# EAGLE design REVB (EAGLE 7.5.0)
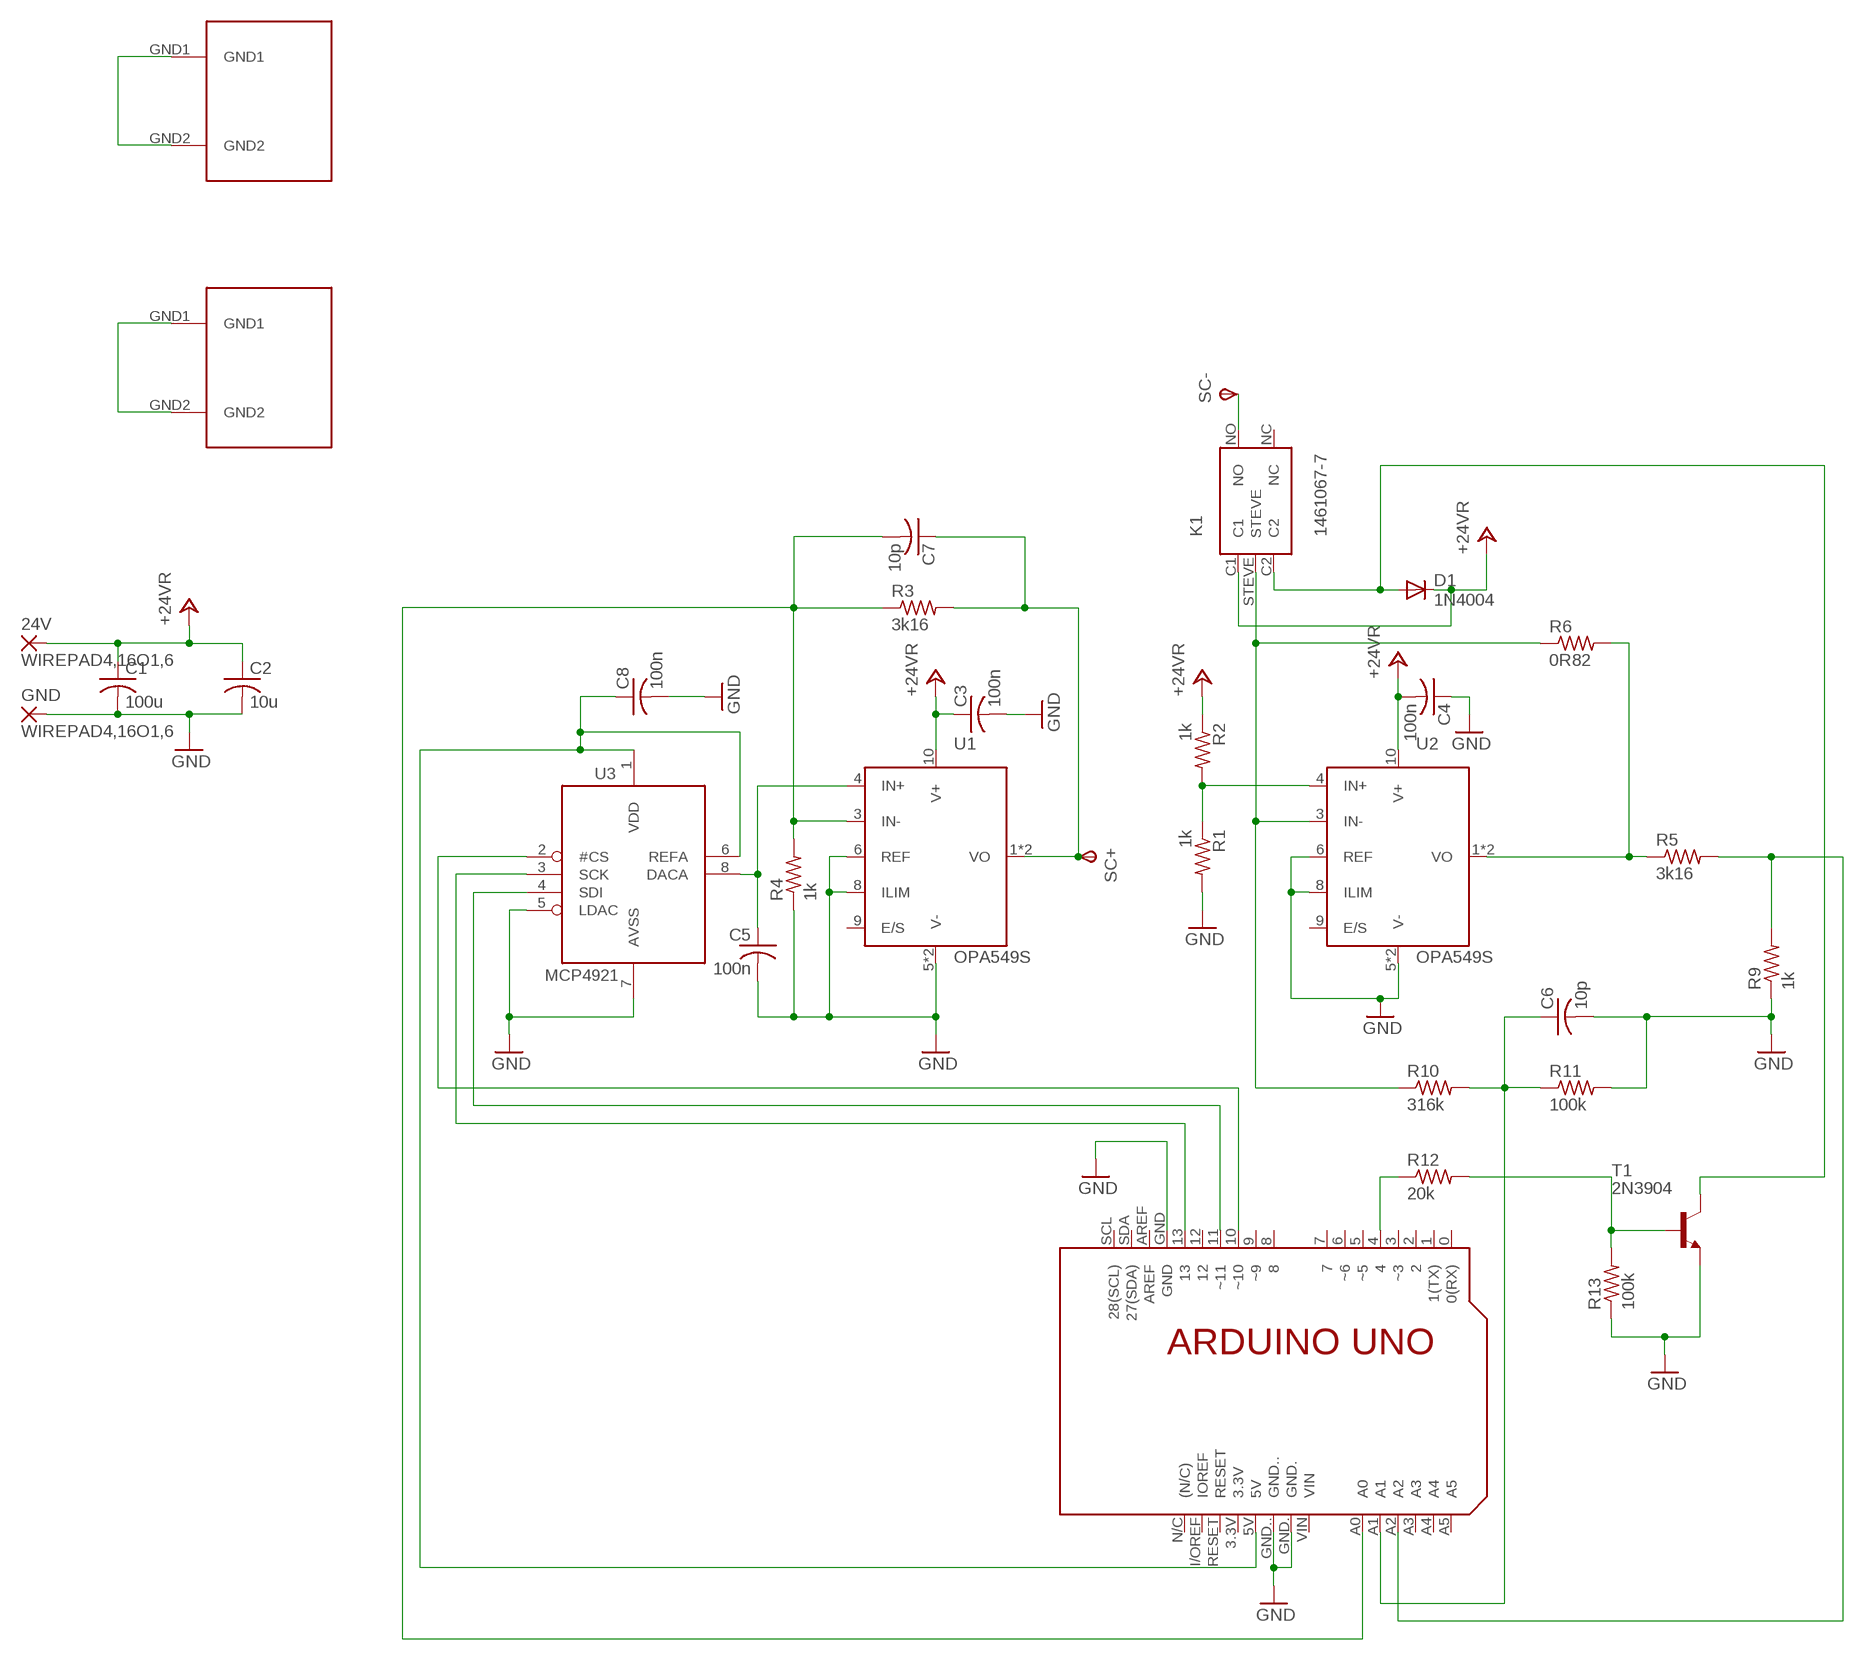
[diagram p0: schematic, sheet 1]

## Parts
24V  WIREPAD4,16O1,6  [4,16O1,6]
C1  100u  C-US050-050X075  [C050-050X075]
C2  10u  C-US025-024X044  [C025-024X044]
C3  100n  C-US025-024X044  [C025-024X044]
C4  100n  C-US025-024X044  [C025-024X044]
C5  100n  C-US025-024X044  [C025-024X044]
C6  10p  C-US025-024X044  [C025-024X044]
C7  10p  C-US025-024X044  [C025-024X044]
C8  100n  C-US025-024X044  [C025-024X044]
D1  1N4004  [DO41-10]
GND  WIREPAD4,16O1,6  [4,16O1,6]
K1  1461067-7  [1461067-7]
PCB1  ARDUINO_UNO  [ARDUINO_UNO]
R1  1k  R-US_0207/10  [0207/10]
R2  1k  R-US_0207/10  [0207/10]
R3  3k16  R-US_0207/10  [0207/10]
R4  1k  R-US_0207/10  [0207/10]
R5  3k16  R-US_0207/10  [0207/10]
R6  0R82  RESHS50  [HS50]
R9  1k  R-US_0207/10  [0207/10]
R10  316k  R-US_0207/10  [0207/10]
R11  100k  R-US_0207/10  [0207/10]
R12  20k  R-US_0207/10  [0207/10]
R13  100k  R-US_0207/10  [0207/10]
SC+  TPSPAD1-20  [P1-20]
SC-  TPSPAD1-20  [P1-20]
T1  2N3904  [TO92]
U1  OPA549S  [11TO-220]
U2  OPA549S  [11TO-220]
U3  MCP4921  [DIL08]
U$7  RA-T2X-64E  [RA-T2X-64E]
U$8  RA-T2X-64E  [RA-T2X-64E]

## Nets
+24V: 24V.1(P) C1.1 C2.1 C3.1 C4.2 D1.C K1.C1 R2.1 U1.10(V+) U2.10(V+) ; supply symbol labelled +24VR
GND: C1.2 C2.2 C3.2 C4.1 C5.2 C6.2 C8.2 GND.1(P) PCB1.GND PCB1.GND. PCB1.GND.. R1.2 R4.1 R9.1 R11.2 R13.1 T1.3(E) U1.5(V-) U1.6(REF) U1.7(V-) U1.8(ILIM) U2.5(V-) U2.6(REF) U2.7(V-) U2.8(ILIM) U3.5(LDAC) U3.7(AVSS)
ISO1: U$8.GND1 U$8.GND2
ISO2: U$7.GND1 U$7.GND2
N$1: C7.1 R3.2 SC+.TP(PP) U1.1(VO) U1.2(VO)
N$2: PCB1.10(~10) U3.2(#CS)
N$3: PCB1.13 U3.3(SCK)
N$4: PCB1.11(~11) U3.4(SDI)
N$5: R5.1 R6.P2 U2.1(VO) U2.2(VO)
N$6: C5.1 U1.4(IN+) U3.8(DACA)
N$7: C7.2 PCB1.A0 R3.1 R4.2 U1.3(IN-)
N$8: K1.NO SC-.TP(PP)
N$10: PCB1.A2 R5.2 R9.2
N$11: C6.1 PCB1.A1 R10.2 R11.1
N$12: PCB1.4 R12.1
N$13: R12.2 R13.2 T1.2(B)
N$14: D1.A K1.C2 T1.1(C)
N$26: K1.STEVE R6.P1 R10.1 U2.3(IN-)
N$31: R1.1 R2.2 U2.4(IN+)
VDD: C8.1 PCB1.5V U3.1(VDD) U3.6(REFA)
Unconnected: K1.NC PCB1.0(0(RX)) PCB1.1(1(TX)) PCB1.2 PCB1.3(~3) PCB1.3.3V PCB1.5(~5) PCB1.6(~6) PCB1.7 PCB1.8 PCB1.9(~9) PCB1.12 PCB1.A3 PCB1.A4 PCB1.A5 PCB1.AREF PCB1.I/OREF(IOREF) PCB1.N/C((N/C)) PCB1.RESET PCB1.SCL(28(SCL)) PCB1.SDA(27(SDA)) PCB1.VIN U1.9(E/S) U2.9(E/S)

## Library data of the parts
24V GND = wirepad:WIREPAD: Wire PAD connect wire on PCB
C1-C8 = rcl:C-US: CAPACITOR, American symbol
D1 = diode:1N4004: DIODE
K1 = aaron:1461067-7
PCB1 = E14_Arduino_revB:ARDUINO_UNO: Device for representing an Arduino Uno board with a footprint in an EAGLE design. Created by Dave Young for Element14. More EAGLE documentation at: http://www.element14.com/community/community/knode/cadsoft_eagle
R1-R5 R9-R13 = resistor:R-US_: RESISTOR, American symbol
R6 = aaron:RES
SC+ SC- = testpad:TPS: TEST PIN
T1 = transistor:2N3904: NPN TRANSISTOR
U1 U2 = aaron:OPA549S
U3 = adafruit:MCP4921
U$7 U$8 = DanECE4901:RA-T2X-64E

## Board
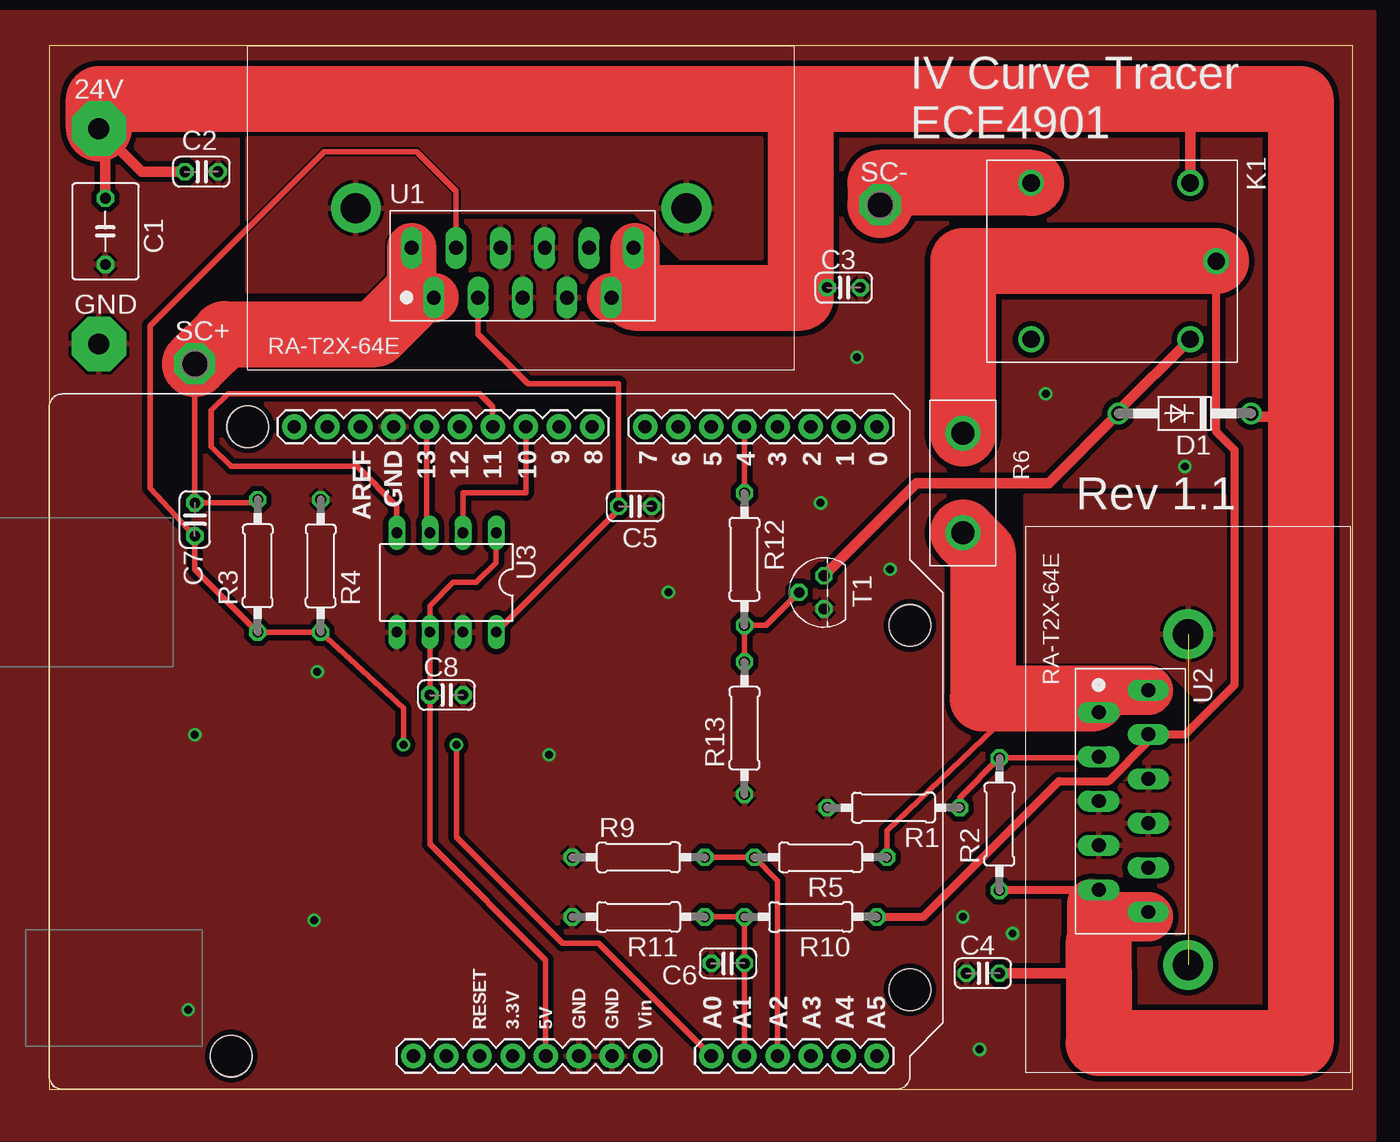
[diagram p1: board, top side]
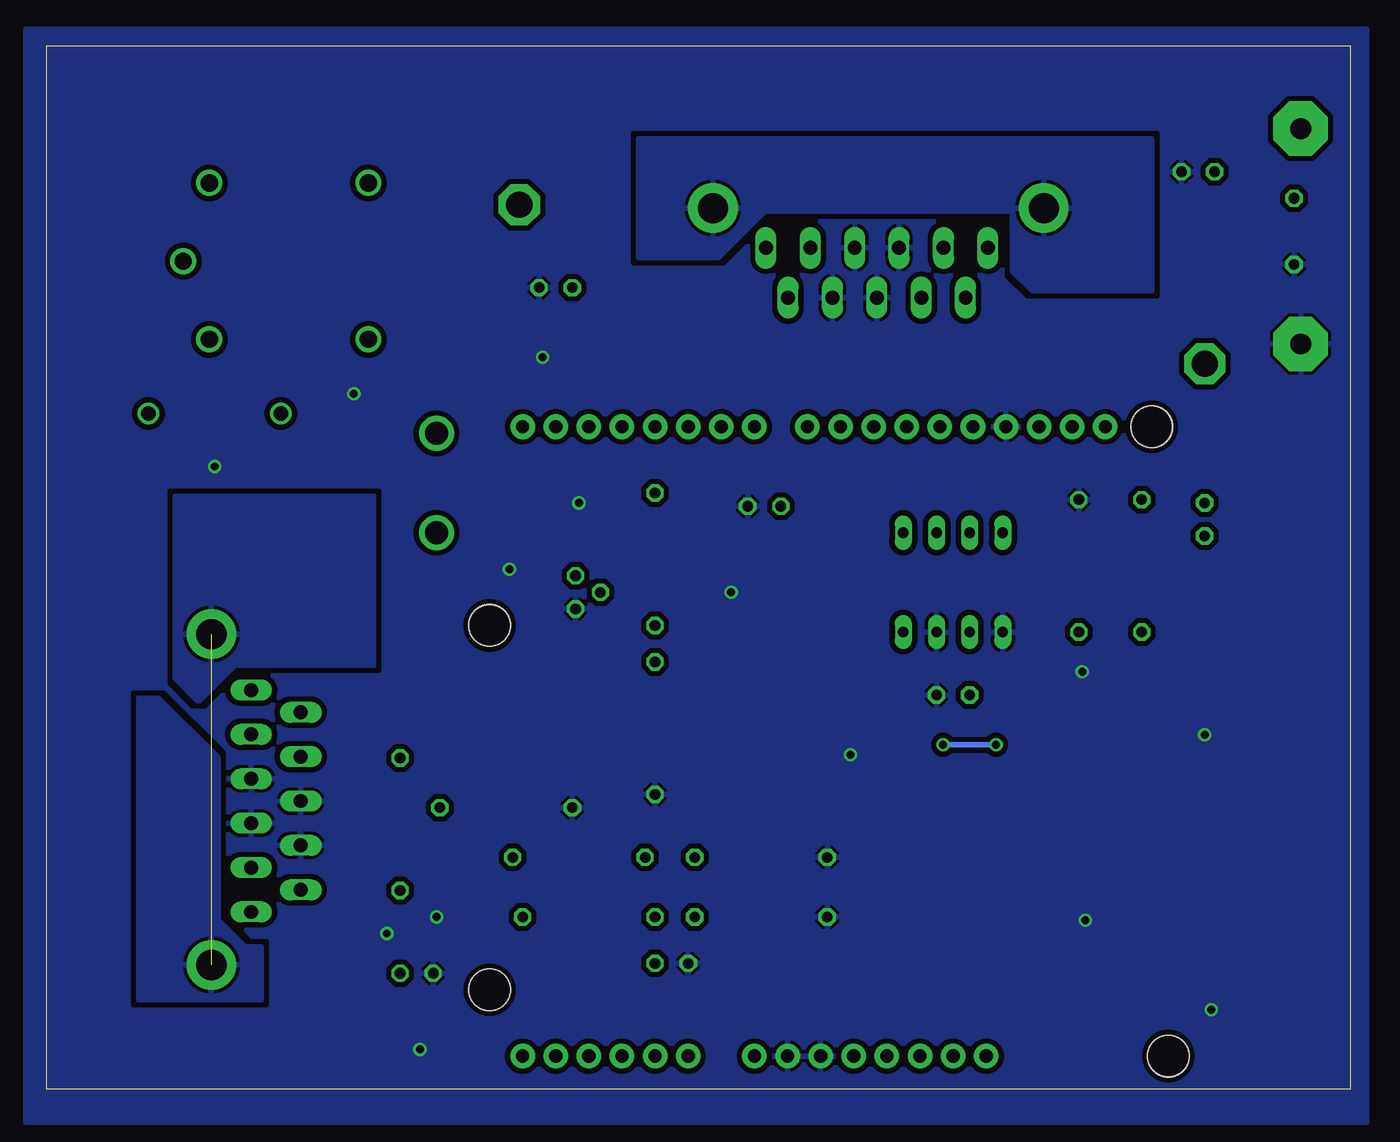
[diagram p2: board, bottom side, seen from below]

No outline drawn. Coordinates in mm, seen from the top.
Copper layers (1*16): Top 0.035559375mm / dielectric 1.501140625mm / Bottom 0.035559375mm
Design rules "typical_4pcb": minimum track width 10mil, minimum drill 15mil, track to track 6mil, track to pad 6mil, pad to pad 6mil, via to via 6mil, smd to smd 6mil, copper to edge 15mil, drill to drill 8mil, minimum pad ring 10mil, minimum via ring 8mil, stop-mask expansion 4mil, vias tented up to drill 0mil, thermal gap 10mil
Holes 3.17 mm at 15.24,50.8 66.04,35.56 66.04,7.62 13.97,2.54
Milling: 4 lines

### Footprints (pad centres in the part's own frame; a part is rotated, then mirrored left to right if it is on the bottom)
4,16O1,6 = drill 1.6 pad 4.166 octagon: 1 0,0
C050-050X075 = drill 0.813 octagon: 1 -2.54,0; 2 2.54,0
C025-024X044 = drill 0.813 octagon: 1 -1.27,0; 2 1.27,0
DO41-10 = drill 1.118: A 5.08,0; C -5.08,0
1461067-7 = drill 1.321: C1 6,6; C2 6,-6; NC -6.2,-6; NO -6.2,6; STEVE 8,0
ARDUINO_UNO = drill 1.016 pad 1.88: 0 63.5,50.8; 1 60.96,50.8; 2 58.42,50.8; 3 55.88,50.8; 3.3V 35.56,2.54; 4 53.34,50.8; 5 50.8,50.8; 5V 38.1,2.54; 6 48.26,50.8; 7 45.72,50.8; 8 41.656,50.8; 9 39.116,50.8; 10 36.576,50.8; 11 34.036,50.8; 12 31.496,50.8; 13 28.956,50.8; A0 50.8,2.54; A1 53.34,2.54; A2 55.88,2.54; A3 58.42,2.54; A4 60.96,2.54; A5 63.5,2.54; AREF 23.876,50.8; GND 26.416,50.8; GND. 43.18,2.54; GND.. 40.64,2.54; I/OREF 30.48,2.54; N/C 27.94,2.54; RESET 33.02,2.54; SCL 18.796,50.8; SDA 21.336,50.8; VIN 45.72,2.54 | hole 3.2: 66.04,7.62; 66.04,35.56; 15.24,50.8; 13.97,2.54
0207/10 = drill 0.813 octagon: 1 -5.08,0; 2 5.08,0
HS50 = drill 1.778: P1 -3.81,0; P2 3.81,0
P1-20 = drill 2.007 pad 3.15 octagon: TP 0,0
TO92 = drill 0.813 octagon: 1 1.27,0; 2 0,1.905; 3 -1.27,0
11TO-220 = drill 1.067 long: 1 -8.509,0; 2 -6.807,-3.81; 3 -5.105,0; 4 -3.404,-3.81; 5 -1.702,0; 6 0,-3.81; 7 1.702,0; 8 3.404,-3.81; 9 5.105,0; 10 6.807,-3.81; 11 8.509,0
DIL08 = drill 0.813 long: 1 -3.81,-3.81; 2 -1.27,-3.81; 3 1.27,-3.81; 4 3.81,-3.81; 5 3.81,3.81; 6 1.27,3.81; 7 -1.27,3.81; 8 -3.81,3.81
RA-T2X-64E = drill 2.311 pad 3.81: GND1 8.28,12.446; GND2 33.655,12.446

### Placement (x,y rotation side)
24V  3.81,73.66 0 top
C1  4.32,65.79 270 top
C2  11.68,70.36 0 top
C3  60.96,61.47 0 top
C4  71.63,8.89 0 top
C5  44.96,44.7 0 top
C6  52.07,9.65 180 top
C7  11.18,43.69 270 top
C8  30.48,30.23 0 top
D1  87.12,51.82 180 top
GND  3.81,57.15 0 top
K1  81.53,63.5 0 top
PCB1  0,0 0 top
R1  64.77,21.59 180 top
R2  72.9,20.32 90 top
R3  16,40.13 90 top
R4  20.83,40.13 270 top
R5  59.18,17.78 180 top
R6  70.1,46.48 270 top
R9  45.21,17.78 0 top
R10  58.42,13.21 180 top
R11  45.21,13.21 180 top
R12  53.34,40.64 270 top
R13  53.34,27.69 90 top
SC+  11.18,55.63 0 top
SC-  63.75,67.82 0 top
T1  59.44,38.1 90 top
U1  36.32,64.52 0 top
U2  84.33,22.1 270 top
U3  30.48,38.86 180 top
U$7  74.93,43.18 270 top
U$8  15.24,55.12 0 top

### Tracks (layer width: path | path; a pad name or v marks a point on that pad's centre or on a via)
+24V
  Top 0.305: 80.01,14.22 80.52,14.73 U2.10
  Top 0.406: 80.01,8.89 80.52,8.89 80.52,9.14 | 87.63,74.42 87.63,75.95
  Top 0.61: 57.66,60.71 58.93,60.71 C3.1 57.4,63.75 57.4,75.95 | R2.1 72.95,15.29 U2.10
  Top 0.813: C4.2 80.01,8.89 | D1.C 92.2,51.56 96.01,51.56 | 3.3,73.15 24V.1 | C1.1 4.32,73.15 24V.1 | C2.1 7.11,70.36 24V.1 | K1.C1 87.53,75.95 88.14,75.95
  Top 3.81: U1.10 44.96,60.71 44.96,64.52 | 80.52,11.18 80.01,11.68 80.01,14.22 81.03,13.21 84.33,13.21
  Top 5.08: 24V.1 3.81,75.95 57.4,75.95 87.63,75.95 88.14,75.95 96.01,75.95 96.01,51.56 96.01,3.56 80.52,3.56 80.52,9.14 80.52,11.18 | 44.96,60.71 57.66,60.71 57.66,73.91
GND  (via drill 0.6, 0.61)
  other vias: 87.12,47.75 11.18,27.18 20.32,12.95 10.67,6.1 47.5,38.1 38.35,25.65 70.1,13.21 73.91,11.94 76.45,53.34 59.18,44.96 64.52,39.88 71.37,3.05 20.57,32 61.98,56.13
  pour Top (isolate 0.406, rank 3): -3.81,82.55 101.6,82.55 101.6,-3.81 -3.81,-3.81
  pour Bottom (isolate 0.406, rank 3): -1.27,81.28 101.6,81.28 101.6,-2.54 -1.27,-2.54
ISO1
  pour Bottom: 54.61,72.9 15.24,72.9 15.24,61.21 24.38,61.21 25.91,62.74 25.91,67.31 44.96,67.31 48.51,63.75 54.61,63.75
  pour Top: 54.61,72.9 15.24,72.9 15.24,61.21 24.38,61.21 25.91,62.74 25.91,67.31 44.96,67.31 48.51,63.75 54.61,63.75
ISO2  (1 unrouted)
  pour Bottom: 90.17,45.47 74.93,45.47 74.93,32.51 85.6,32.51 88.39,29.72 90.17,31.5
  pour Top: 90.17,45.47 74.93,45.47 74.93,32.51 85.6,32.51 88.39,29.72 90.17,31.5
  pour Bottom: 83.57,6.86 92.96,6.86 92.96,29.97 91.44,29.97 86.87,25.4 86.87,12.95 84.84,10.92 83.57,10.92
N$1
  Top 0.406: R3.2 16,44.96 C7.1 SC+.TP
  Top 3.81: U1.1 27.81,60.71 U1.2
  Top 5.08: SC+.TP 13.46,57.91 25.02,57.91 27.81,60.71
N$2
  Top 0.406: PCB1.10 36.58,45.72 31.75,45.72 U3.2
N$3
  Top 0.406: PCB1.13 28.96,42.67 U3.3
N$4
  Top 0.406: PCB1.11 34.04,52.32 33.02,53.34 13.72,53.34 12.45,52.07 12.45,49.28 13.97,47.75 23.62,47.75 26.67,44.7 U3.4
N$5
  Top 0.406: R5.1 64.26,19.81 74.93,29.97
  Top 1.778: U2.2 80.52,30.48 | 80.52,30.48 79.5,30.61 | 80.01,29.97 79.5,30.48 80.52,30.48
  Top 3.81: U2.1 79.5,30.61
  Top 5.08: R6.P2 71.63,41.15 71.63,29.97 74.93,29.97 80.01,29.97
N$6
  Top 0.406: U3.8 43.69,44.45 C5.1 43.69,54.1 36.73,54.1 32.92,57.91 U1.4
N$7  (via drill 0.61)
  Top 0.406: PCB1.A0 42.16,11.18 39.37,11.18 31.24,19.3 v31.24,26.42 | U1.3 31.22,68.86 28.19,71.88 21.08,71.88 7.75,58.55 7.75,46.1 C7.2 11.18,39.88 R3.1 R4.2 27.18,29.21 v27.18,26.42
  Bottom 0.406: v31.24,26.42 v27.18,26.42
N$8
  Top 5.08: K1.NO 63.75,69.5 SC-.TP
N$10
  Top 0.406: R9.2 R5.2 55.88,16 PCB1.A2
N$11
  Top 0.406: R11.1 R10.2 C6.1 PCB1.A1
N$12
  Top 0.406: PCB1.4 R12.1
N$13
  Top 0.406: R13.2 R12.2 54.99,35.56 T1.2
N$14
  Top 0.813: K1.C2 82.04,52.01 D1.A 76.71,46.48 66.55,46.48 T1.1
N$26
  Top 0.61: R10.1 67.06,13.21 77.47,23.62 81.28,23.62 84.33,26.67 U2.3 87.15,27.2 90.93,30.99 90.93,49.02 89.53,50.42 K1.STEVE
  Top 5.08: K1.STEVE 70.1,63.5 R6.P1
N$31
  Top 0.406: R1.1 69.85,22.35 R2.2 80.42,25.4 U2.4
VDD
  Top 0.406: PCB1.5V 38.1,9.91 29.21,18.8 C8.1 U3.6 29.21,37.08 30.99,38.86 32.77,38.86 34.29,40.39 U3.1

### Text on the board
tPlace: IV Curve Tracer / ECE4901 | Rev 1.1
